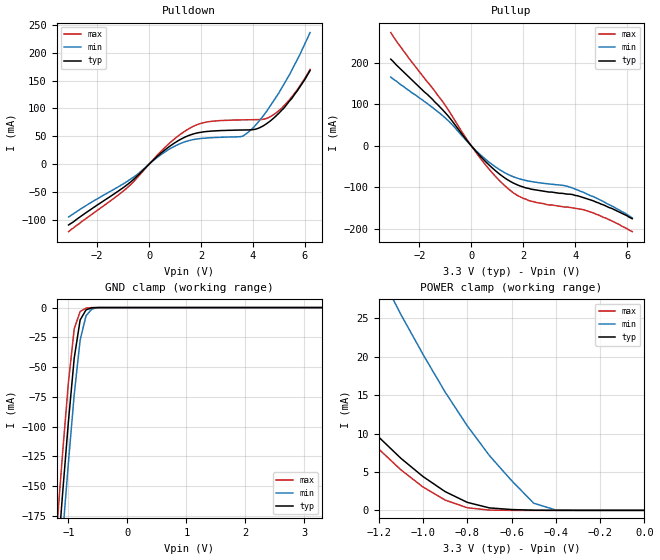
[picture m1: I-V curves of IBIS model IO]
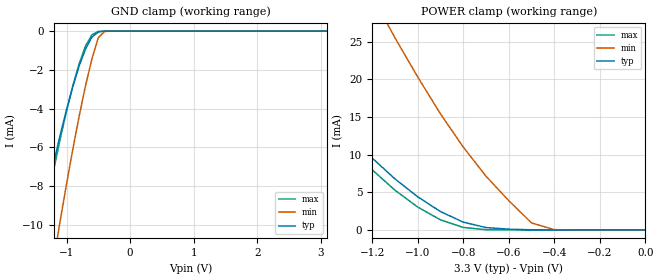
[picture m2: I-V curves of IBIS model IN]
[IBIS Ver]   1.1
[File name]   69d536.ibs
[File Rev]   1.0
[Date]   8/19/98
[Source]   This file originated at Motorola Fast SRAM.
[Notes]
1. This I/O model good for MCM69D536 & MCM69D618.
[Disclaimer]   Data is for modeling purposes only and is not guaranteed
[Component]   32Kx36 & 64Kx18 1Mb NetRAM.
[Manufacturer] Motorola
[Package]
|  RLC Data is subject to change after further study of package
|		typ		min		max
R_pkg		200m		150m		250m
L_pkg		5.5nH		4nH		7nH
C_pkg		2pF		1.5pF		2.5pF
[Pin]		signal_name	model_name	R_pin		L_pin		C_pin
1		VSS		GND		NA		NA		NA
2		DQX20		IO		NA		NA		NA
3		DQY20		IO		NA		NA		NA
4		VDD		POWER		NA		NA		NA
5		VSS		GND		NA		NA		NA
6		DQX21		IO		NA		NA		NA
7		DCY21		IO		NA		NA		NA
8		DQX22		IO		NA		NA		NA
9		DQY22		IO		NA		NA		NA
10		VDD		POWER		NA		NA		NA
11		VSS		GND		NA		NA		NA
12		DQX23		IO		NA		NA		NA
13		DQY23		IO		NA		NA		NA
14		DQX24		IO		NA		NA		NA
15		DQY24		IO		NA		NA		NA
16		VDD		POWER		NA		NA		NA
17		VSS		GND		NA		NA		NA
18		DQX25		IO		NA		NA		NA
19		DQY25	 	IO		NA		NA		NA
20		DQX26		IO		NA		NA		NA
21		DQY26		IO		NA		NA		NA
22		VDD		POWER		NA		NA		NA
23		VSS		GND		NA		NA		NA
24		DQY27		IO		NA		NA		NA
25		DQX27		IO		NA		NA		NA
26		DQY28		IO		NA		NA		NA
27		DQX28		IO		NA		NA		NA
28		VDD		POWER		NA		NA		NA
29		VSS		GND		NA		NA		NA
30		DQY29		IO		NA		NA		NA
31		DQX29		IO		NA		NA		NA
32		DQY30		IO		NA		NA		NA
33		DQX30		IO		NA		NA		NA
34		VDD		POWER		NA		NA		NA
35		VSS		GND		NA		NA		NA
36		DQY31		IO		NA		NA		NA
37		DQX31		IO		NA		NA		NA
38		DQY32		IO		NA		NA		NA
39		DQX32		IO		NA		NA		NA
40		VDD		POWER		NA		NA		NA
41		VSS		GND		NA		NA		NA
42		DQY33		IO		NA		NA		NA
43		DQX33		IO		NA		NA		NA
44		VSS		GND		NA		NA		NA
45		VSS		GND		NA		NA		NA
46		DQY34		IO		NA		NA		NA
47		DQX34		IO		NA		NA		NA
48		VSS		GND		NA		NA		NA
49		VDD		POWER		NA		NA		NA
50		DQY35		IO		NA		NA		NA
51		DQX35		IO		NA		NA		NA
52		VSS		GND		NA		NA		NA
53		VSS		GND		NA		NA		NA
54		AY5		IN		NA		NA		NA
55		AX5		IN		NA		NA		NA
56		AY4		IN		NA		NA		NA
57		AX4		IN		NA		NA		NA
58		AY3		IN		NA		NA		NA
59		AX3		IN		NA		NA		NA
60		AY2		IN		NA		NA		NA
61		AX2		IN		NA		NA		NA
62		AY1		IN		NA		NA		NA
63		AX1		IN		NA		NA		NA
64		AY0		IN		NA		NA		NA
65		AX0		IN		NA		NA		NA
66		VSS		GND		NA		NA		NA
67		VDD		POWER		NA		NA		NA
68		AX10		IN		NA		NA		NA
69		AY10		IN		NA		NA		NA
70		AX11		IN		NA		NA		NA
71		AY11		IN		NA		NA		NA
72		AX12		IN		NA		NA		NA
73		AY12		IN		NA		NA		NA
74		AX13		IN		NA		NA		NA
75		AY13		IN		NA		NA		NA
76		AX14		IN		NA		NA		NA
77		AY14		IN		NA		NA		NA
78		NC		NC		NA		NA		NA
79		NC		NC		NA		NA		NA
80		NC		NC		NA		NA		NA
81		NC		NC		NA		NA		NA
82		DQX0		IO		NA		NA		NA
83		DQY0		IO		NA		NA		NA
84		VDD		POWER		NA		NA		NA
85		VSS		GND		NA		NA		NA
86		DQX1		IO		NA		NA		NA
87		DQY1		IO		NA		NA		NA
88		VSS		GND		NA		NA		NA
89		VSS		GND		NA		NA		NA
90		DQX2		IO		NA		NA		NA
91		DQY2		IO		NA		NA		NA
92		VDD		POWER		NA		NA		NA
93		VSS		GND		NA		NA		NA
94		DQX3		IO		NA		NA		NA
95		DQY3		IO		NA		NA		NA
96		DQX4		IO		NA		NA		NA
97		DQY4		IO		NA		NA		NA
98		VDD		POWER		NA		NA		NA
99		VSS		GND		NA		NA		NA
100		DQX5		IO		NA		NA		NA
101		DQY5		IO		NA		NA		NA
102		DQX6		IO		NA		NA		NA
103		DQY6		IO		NA		NA		NA
104		VDD		POWER		NA		NA		NA
105		VSS		GND		NA		NA		NA
106		DQX7		IO		NA		NA		NA
107		DQY7		IO		NA		NA		NA
108		DQX8		IO		NA		NA		NA
109		DQY8		IO		NA		NA		NA
110		VDD		POWER		NA		NA		NA
111		VSS		GND		NA		NA		NA
112		DQY9		IO		NA		NA		NA
113		DQX9		IO		NA		NA		NA
114		DQY10		IO		NA		NA		NA
115		DQX10		IO		NA		NA		NA
116		VDD		POWER		NA		NA		NA
117		VSS		GND		NA		NA		NA
118		DQY11		IO		NA		NA		NA
119		DQX11	 	IO		NA		NA		NA
120		DQY12		IO		NA		NA		NA
121		DQX12		IO		NA		NA		NA
122		VDD		POWER		NA		NA		NA
123		VSS		GND		NA		NA		NA
124		DQY13		IO		NA		NA		NA
125		DQX13		IO		NA		NA		NA
126		DQY14		IO		NA		NA		NA
127		DQX14		IO		NA		NA		NA
128		VDD		POWER		NA		NA		NA
129		VSS		GND		NA		NA		NA
130		DQY15		IO		NA		NA		NA
131		DQX15		IO		NA		NA		NA
132		VSS		GND		NA		NA		NA
133		VSS		GND		NA		NA		NA
134		DQY16		IO		NA		NA		NA
135		DQX16		IO		NA		NA		NA
136		VSS		GND		NA		NA		NA
137		VDD		POWER		NA		NA		NA
138		DQY17		IO		NA		NA		NA
139		DQX17		IO		NA		NA		NA
140		NC		NC		NA		NA		NA
141		NC		NC		NA		NA		NA
142		AY9		IN		NA		NA		NA
143		AX9		IN		NA		NA		NA
144		AY8		IN		NA		NA		NA
145		AX8		IN		NA		NA		NA
146		PTX#		IN		NA		NA		NA
147		PTY#		IN		NA		NA		NA
148		WX#		IN		NA		NA		NA
149		WY#		IN		NA		NA		NA
150		E1#		IN		NA		NA		NA
151		E2		IN		NA		NA		NA
152		GX#		IN		NA		NA		NA
153		GY#		IN		NA		NA		NA
154		VSS		GND		NA		NA		NA
155		VDD		POWER		NA		NA		NA
156		K		IN		NA		NA		NA
157		NC		NC		NA		NA		NA
158		NC		NC		NA		NA		NA
159		NC		NC		NA		NA		NA
160		NC		NC		NA		NA		NA
161		NC		NC		NA		NA		NA
162		NC		NC		NA		NA		NA
163		NC		NC		NA		NA		NA
164		NC		NC		NA		NA		NA
165		VSS		GND		NA		NA		NA
166		AY7		IN		NA		NA		NA
167		AX7		IN		NA		NA		NA
168		AY6		IN		NA		NA		NA
169		AX6		IN		NA		NA		NA
170		DQX18		IO		NA		NA		NA
171		DQY18		IO		NA		NA		NA
172		VDD		POWER		NA		NA		NA
173		VSS		GND		NA		NA		NA
174		DQX19		IO		NA		NA		NA
175		DQY19		IO		NA		NA		NA
176		VSS		GND		NA		NA		NA
| Models and submodels in the file (2): IO (I/O), IN (Input)
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| BI-DIRECTIONAL I/O MODEL
[Model]   IO
Model_type  I/O
Polarity   Non-Inverting
Enable   Active-Low
|signals  DQX, DQY
|Variable   typ   min   max
C_comp   6pF   NA   8pF
|Variable   typ   min   max
[Voltage range]   3.3   3.1  3.6
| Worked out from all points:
|   slope of the pulldown table from 0 to 0.495 V, typ, clamps not added: 23.3 ohm
|   slope of the pullup table from 0 to 0.495 V, typ, clamps not added: 14.4 ohm
|   GND clamp passes 1 mA (typ) near -0.65 V on its own axis
|   POWER clamp passes 1 mA (typ) near -0.79 V on its own axis
|Temp used   50C   100C   0C
|Variable   typ   min   max
|NOTE: All V/I tables should have at least 3 entries.
|   0.0 volts, 2*supply_voltage and -supply_voltage
[Pulldown]
|Volt	Typical		Minimum		Maximum
-3.1V     -109mA     -94.7mA    -121mA
-900mV    -38.8mA    -32.6mA    -44.6mA
500mV     21.4mA     18.4mA     25mA
1.4V      48.9mA     40.4mA     59.8mA
2.2V      58.5mA     46.8mA     75.4mA
3.5V      61.2mA     49.2mA     79.3mA
3.8V      61.4mA     56.5mA     79.6mA
4.3V      66.3mA     81mA       80mA
4.6V      75.1mA     99.8mA     83.5mA
4.9V      87mA       121mA      92.3mA
5.4V      113mA      160mA      115mA
6.2V      168mA      236mA      170mA
[Pullup]
|Volt	Typical		Minimum		Maximum
-3.1V     208mA      165mA      272mA
-2.4V     165mA      133mA      210mA
-1.1V     86.2mA     72.2mA     106mA
-200mV    15.4mA     13.3mA     18.3mA
300mV     -21.4mA    -18.4mA    -25.8mA
900mV     -58.1mA    -49.2mA    -71.3mA
1.4V      -81.6mA    -68.2mA    -102mA
1.8V      -94.4mA    -78.2mA    -120mA
2.3V      -104mA     -85.6mA    -133mA
3.9V      -117mA     -101mA     -149mA
4.7V      -132mA     -122mA     -161mA
6.2V      -175mA     -173mA     -206mA
[GND_clamp]
|Volt	Typical		Minimum	Maximum
-3.3V     -2.318A    -2.336A    -2.303A
-1.2V     -223mA     -258mA     -189mA
-1.1V     -158mA     -193mA     -124mA
-1V       -96.5mA    -131mA     -63.6mA
-900mV    -42.3mA    -72.9mA    -17.8mA
-800mV    -10.4mA    -27.2mA    -3.33mA
-700mV    -1.94mA    -6.83mA    -442uA
-600mV    -175uA     -1.16mA    -23.1uA
-500mV    -7.07uA    -76.7uA    -1.47uA
3.3V      59.7pA     95.9pA     59.4pA
[POWER_clamp]
|Volt	Typical		Minimum		Maximum
-3.1V     105mA      173mA      110mA
-1.7V     27.7mA     62.5mA     26.7mA
-1.6V     23.6mA     55.8mA     22.4mA
-1.4V     16mA       43mA       14.5mA
-1.2V     9.54mA     31.1mA     7.98mA
-1.1V     6.78mA     25.5mA     5.28mA
-900mV    2.44mA     15.4mA     1.34mA
-800mV    1.04mA     11mA       338uA
-700mV    319uA      7.13mA     33.9uA
-500mV    20.9uA     933uA      150nA
-400mV    578nA      41.7uA     2.74nA
0V        469pA      626pA      504pA
[Ramp]
|Variable   typ   min	max
dV/dt_r  1.50/0.33n	NA	NA
dV/dt_f  1.29/0.13n	NA	NA
| STANDARD INPUT MODEL
[Model]   IN
Model_type  Input
Polarity   Non-Inverting
|signals  GX/Y#, K, AX, AY, PTX#, PTY#, E1#, E2, WX#, WY#|
|Variable   typ   min   max
C_comp   4pF   NA   5pF
|Variable   typ   min   max
[Voltage range]   3.3   3.1  3.6
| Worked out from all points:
|   GND clamp passes 1 mA (typ) near -0.71 V on its own axis
|   POWER clamp passes 1 mA (typ) near -0.79 V on its own axis
|Temp used   50C   100C   0C
[GND_clamp]
|Volt	Typical		Minimum		Maximum
-3.1V     -45.8mA    -60.1mA    -49.3mA
-1.5V     -11.5mA    -18.1mA    -12.3mA
-1.4V     -9.83mA    -15.9mA    -10.5mA
-1.2V     -6.78mA    -11.8mA    -7.13mA
-1.1V     -5.37mA    -9.8mA     -5.57mA
-900mV    -2.86mA    -6.08mA    -2.81mA
-800mV    -1.79mA    -4.37mA    -1.67mA
-700mV    -918uA     -2.8mA     -759uA
-600mV    -310uA     -1.43mA    -192uA
-500mV    -48.2uA    -340uA     -17.7uA
-300mV    -165nA     -1.28uA    -19.6nA
3.1V      425pA      626pA      394pA
[POWER_clamp]
|Volt	Typical		Minimum		Maximum
-3.1V     105mA      173mA      110mA
-1.7V     27.7mA     62.5mA     26.7mA
-1.6V     23.6mA     55.8mA     22.4mA
-1.4V     16mA       43mA       14.5mA
-1.2V     9.54mA     31.1mA     7.98mA
-1.1V     6.78mA     25.5mA     5.28mA
-900mV    2.44mA     15.4mA     1.34mA
-800mV    1.04mA     11mA       338uA
-700mV    319uA      7.13mA     33.9uA
-500mV    20.9uA     933uA      150nA
-400mV    578nA      41.7uA     2.74nA
0V        469pA      626pA      504pA
